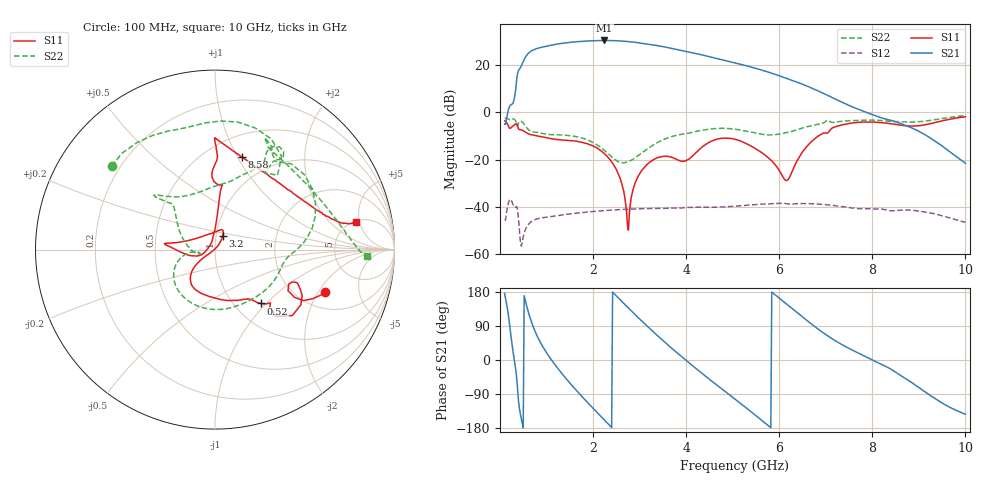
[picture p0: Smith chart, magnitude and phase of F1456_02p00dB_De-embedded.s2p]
! Integrated Device Technology
! Corporate Headquarters
! 6024 Silver Creek Valley Road
! San Jose, CA 95138  USA
! Phone:  1-408-284-8200
! Toll Free:  1-800-223-1366
! Webpage:  http://www.idt.com/
! Timing and RF Division
! 515 Groton Road, Suite 102
! Westford, MA 01886-6024
! Device:  F1456
! Description: 6-bit 0.5 dB Transmit Variable Gain Amplifier
! Frequency:  2100.0 -  2950.00 MHz
! Package:  6x6 mm Thin QFN Plastic Package: 28 pin
! State:  4
! Atten State:  2.0 dB
! Voltage:  +5.00 Volts
! Current:  214.093 mA
! Data:  The device was measured on a the F1455 evaluation board which has
!  individual transmission lines to the RF pins.  Data was collected
!  using a calibrated network analyzer.  The evaluation board was
!  de-embedded using a TRL calibration technique.
!  The reference plane is the edge of the package pin.
!  Pin  1 = CSb
!  Pin  2 = DATA
!  Pin  3 = CLK
!  Pin  4 = RSET
!  Pin  5 = GND
!  Pin  6 = RFIN  = Port 1
!  Pin  7 = GND
!  Pin  8 = NC
!  Pin  9 = NC
!  Pin 10 = NC
!  Pin 11 = NC
!  Pin 12 = NC
!  Pin 13 = NC
!  Pin 14 = /STBY
!  Pin 15 = GND
!  Pin 16 = RFOUT  = Port 2
!  Pin 17 = GND
!  Pin 18 = NC
!  Pin 19 = NC
!  Pin 20 = NC
!  Pin 21 = GND
!  Pin 22 = NC
!  Pin 23 = GND
!  Pin 24 = NC
!  Pin 25 = NC
!  Pin 26 = NC
!  Pin 27 = GND
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# GHz S dB R 50
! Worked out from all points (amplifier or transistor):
!   496 points, 100 MHz to 10 GHz, reference 50 ohm
!   highest |S21| = 30.3 dB at 2.24 GHz (marker M1)
!   |S21| within 3 dB of that: 870.3 MHz to 3.607 GHz (2.736 GHz wide, 122 % of centre)
!   unconditionally stable (mu >= 1): start of sweep to end of sweep
!   at 1.74 GHz: K = 2.02, MAG = 30.4 dB, |S12| = -42.4 dB
!   at 5.06 GHz: K = 3.50, MAG = 21.8 dB, |S12| = -39.6 dB
!   at 10 GHz: K = 130.93, MAG = -11.7 dB, |S12| = -46.5 dB
!   S11 on the Smith chart (normalised r, x): 100 MHz: 2.75, -2.29; 520 MHz: 1.31, -0.93; 3.2 GHz: 1.08, +0.16; 8.58 GHz: 0.72, +1.04; 10 GHz: 5.12, +4.43
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0.1  -3.66 -21.2  -5.06 175.6  -45.34 41.8  -2.61 141.1
0.34  -4.90 -32.7  9.95 -25.6  -40.11 -141.8  -3.89 54.5
0.42  -7.35 -43.9  18.13 -128.9  -50.27 137.5  -3.88 48.3
0.52  -8.09 -49.6  22.24 169.9  -51.07 -162.0  -5.11 12.6
0.64  -9.33 -54.3  25.35 114.2  -46.75 162.0  -7.79 -5.9
0.76  -9.89 -59.8  26.62 74.0  -45.31 129.8  -8.45 -20.2
1.12  -11.25 -87.5  28.34 -2.1  -44.05 73.5  -9.48 -73.2
1.46  -11.93 -109.8  29.37 -54.9  -43.02 44.6  -9.81 -115.7
1.76  -12.73 -125.3  29.89 -96.2  -42.36 24.4  -10.90 -143.0
2.24  -17.44 -141.4  30.26 -158.0  -41.52 -3.0  -16.06 -171.9
2.5  -24.16 -145.0  30.14 169.3  -41.21 -16.9  -20.39 -171.5
2.78  -43.05 66.9  29.74 134.7  -40.94 -31.2  -20.70 -164.7
3.2  -21.40 60.4  28.69 85.1  -40.68 -51.9  -15.03 164.7
3.4  -19.15 65.5  28.03 62.4  -40.60 -61.2  -12.66 149.8
3.8  -19.99 86.9  26.49 19.3  -40.49 -78.6  -9.75 134.3
4.3  -15.49 163.6  24.36 -31.2  -40.10 -101.1  -7.79 136.9
5.06  -11.48 175.2  20.73 -104.1  -39.65 -132.6  -7.23 135.9
5.68  -17.84 -164.1  17.43 -164.8  -38.81 -165.3  -9.43 116.4
6.7  -12.30 85.6  10.15 94.2  -38.62 130.8  -5.67 62.2
8.36  -4.77 83.3  -3.25 -21.3  -41.53 56.8  -3.84 62.5
8.58  -5.42 73.9  -4.58 -38.2  -41.39 51.7  -4.05 56.7
10  -1.93 11.2  -21.59 -142.9  -46.52 -24.1  -1.46 -2.5
